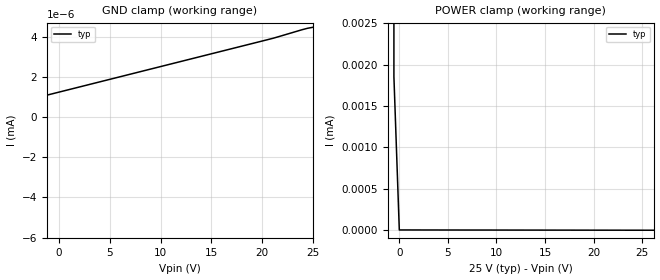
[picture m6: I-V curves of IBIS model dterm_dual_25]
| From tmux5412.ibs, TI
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| dterm_dual_25
[Model]   dterm_dual_25
Model_type   Terminator
|   typ   min   max
C_comp   1.008417e-11   NA   NA
[Voltage Range]   25   NA   NA
[Temperature Range]   27   NA   NA
[Power Clamp Reference]   25   NA   NA
[GND Clamp Reference]   0   NA   NA
[GND Clamp]
|   Voltage   I(typ)   I(min)   I(max)
-30V      -2.839A    NA         NA
-25.56V   -15.04uA   NA         NA
-25V      -1.968nA   NA         NA
-21.11V   -1.44nA    NA         NA
20.56V    3.853nA    NA         NA
25V       4.466nA    NA         NA
[POWER Clamp]
|   Voltage   I(typ)   I(min)   I(max)
-5V       2.611A     NA         NA
-1.111V   49.09mA    NA         NA
-555.6mV  1.854uA    NA         NA
0V        4.466nA    NA         NA
50V       -1.968nA   NA         NA
